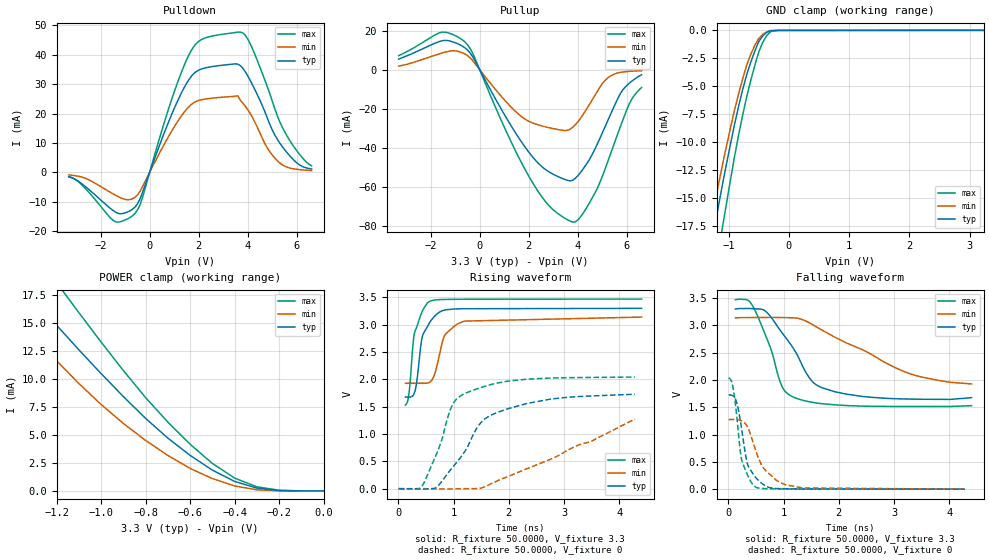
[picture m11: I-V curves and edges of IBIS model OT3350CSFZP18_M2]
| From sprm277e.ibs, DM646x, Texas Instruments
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|   Model Cell OT3350CSFZP18_M2
[Model]   OT3350CSFZP18_M2
Model_type   3-state
Polarity   Non-Inverting
Enable   Active-Low
Cref =  10.0000pF
Rref =  50.0000
Vref =  1.5V
Vmeas =  1.65
C_comp   1.576969p   1.541206p   1.618956p
[Temperature Range]   25   105   0
[Voltage Range]   3.3   3.14   3.47
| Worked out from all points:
|   slope of the pulldown table from 0 to 0.495 V, typ, clamps not added: 44 ohm
|   slope of the pullup table from 0 to 0.495 V, typ, clamps not added: 42.8 ohm
|   GND clamp passes 1 mA (typ) near -0.50 V on its own axis
|   POWER clamp passes 1 mA (typ) near -0.42 V on its own axis
|   rising waveform, R_fixture 50.0000, V_fixture 3.3: 20-80 % time 191ps typ, 250ps min, 163ps max; typ from 1.68 V to 3.3 V
|   rising waveform, R_fixture 50.0000, V_fixture 0: 20-80 % time 815ps typ, 1.73ns min, 454ps max; typ from 0 V to 1.73 V
|   falling waveform, R_fixture 50.0000, V_fixture 3.3: 20-80 % time 603ps typ, 1.42ns min, 389ps max; typ from 3.3 V to 1.68 V
|   falling waveform, R_fixture 50.0000, V_fixture 0: 20-80 % time 210ps typ, 374ps min, 169ps max; typ from 1.73 V to 0 V
[POWER_clamp]
|   voltage   I(typ)   I(min)   I(max)
-3.3V     74.53mA    58.44mA    90.4mA
-1.467V   21.35mA    17.44mA    26.25mA
-1.3V     17.11mA    13.76mA    21.37mA
-1.167V   14.08mA    10.96mA    17.73mA
-1.133V   13.35mA    10.28mA    16.83mA
-1V       10.49mA    7.727mA    13.31mA
-800mV    6.483mA    4.516mA    8.338mA
-600mV    3.176mA    2.013mA    4.168mA
-500mV    1.855mA    1.1mA      2.455mA
-400mV    849.1uA    441.8uA    1.144mA
-300mV    251.7uA    97.47uA    366.8uA
0V        16.5nA     56.13nA    73.26nA
[Pulldown]
|   voltage   I(typ)   I(min)   I(max)
-3.3V     -1.51mA    -878.4uA   -1.475mA
-1.4V     -13.5mA    -7.756mA   -16.81mA
-700mV    -12.57mA   -9.011mA   -14.79mA
-400mV    -9.189mA   -6.568mA   -11.22mA
900mV     19.74mA    14.05mA    24.87mA
1.7V      32.7mA     23.11mA    41.52mA
2.2V      35.39mA    24.85mA    45.53mA
3.6V      36.79mA    25.99mA    47.71mA
4.1V      31.26mA    20mA       43.72mA
5.2V      11.29mA    3.968mA    19.31mA
5.8V      4.81mA     1.296mA    9.68mA
6.6V      1.127mA    609.7uA    2.209mA
[Pullup]
|   voltage   I(typ)   I(min)   I(max)
-3.3V     5.39mA     1.812mA    7.116mA
-1.6V     14.52mA    8.237mA    18.97mA
-600mV    11.14mA    7.957mA    14.14mA
-300mV    6.902mA    4.842mA    8.81mA
1.3V      -29.12mA   -19.41mA   -37.44mA
2.2V      -45.34mA   -27.51mA   -58.77mA
2.9V      -52.9mA    -29.96mA   -70.6mA
3.8V      -56.59mA   -29.42mA   -78.12mA
4.5V      -45.45mA   -17.3mA    -67.66mA
5.2V      -26.73mA   -4.484mA   -47.83mA
6.1V      -6.93mA    -895.9uA   -17.46mA
6.6V      -2.645mA   -585.5uA   -9.164mA
[GND_clamp]
|   voltage   I(typ)   I(min)   I(max)
-3.3V     -90.23mA   -71.94mA   -107.2mA
-1.3V     -19.77mA   -17.29mA   -24.19mA
-1.233V   -17.67mA   -15.49mA   -21.92mA
-1.167V   -15.64mA   -13.72mA   -19.7mA
-1.1V     -13.7mA    -11.97mA   -17.52mA
-900mV    -8.37mA    -7.079mA   -11.23mA
-700mV    -3.966mA   -3.106mA   -5.945mA
-500mV    -1.006mA   -723.8uA   -1.941mA
-366.7mV  -173uA     -140.2uA   -460.9uA
-300mV    -29.43uA   -31.76uA   -99.43uA
-166.7mV  -4.076uA   -4.557uA   -8.063uA
3.233V    -14.06nA   1.378uA    -34.96nA
[Ramp]
| variable   typ   min   max
dV/dt_f  1.0006312/0.62474123n 0.77996615/1.5665136n  1.1807758/0.39522718n
dV/dt_r  1.0444207/0.82282857n 0.78275401/2.2258011n  1.2330064/0.45843701n
R_load = 50
[Rising Waveform]
R_fixture = 50.0000
V_fixture = 3.3
V_fixture_min = 3.14
V_fixture_max = 3.47
|   time   V(typ)   V(min)   V(max)
128.8ps   1.676V     1.928V     1.53V
194.7ps   1.677V     1.929V     1.747V
294ps     1.757V     1.929V     2.847V
336ps     1.964V     1.929V     2.961V
429.8ps   2.756V     1.928V     3.232V
574.4ps   3.05V      1.953V     3.429V
665.6ps   3.164V     2.119V     3.453V
837.5ps   3.268V     2.799V     3.463V
1.197ns   3.293V     3.067V     3.467V
4.402ns   3.3V       3.14V      3.47V
[Rising Waveform]
R_fixture = 50.0000
V_fixture = 0
V_fixture_min = 0
V_fixture_max = 0
|   time   V(typ)   V(min)   V(max)
8.072ps   17.64uV    17.18uV    19.99uV
428.3ps   -8.284mV   14.33uV    42.96mV
687ps     22.56mV    -1.575mV   622mV
965.9ps   369.3mV    -4.262mV   1.503V
1.053ns   475.1mV    -2.583mV   1.637V
1.201ns   675.7mV    -1.005mV   1.739V
1.519ns   1.234V     17.47mV    1.859V
1.971ns   1.458V     217mV      1.965V
2.879ns   1.654V     596mV      2.028V
4.282ns   1.728V     1.275V     2.043V
[Falling Waveform]
R_fixture = 50.0000
V_fixture = 3.3
V_fixture_min = 3.14
V_fixture_max = 3.47
|   time   V(typ)   V(min)   V(max)
128.8ps   3.3V       3.14V      3.47V
337.5ps   3.31V      3.143V     3.469V
433.7ps   3.307V     3.144V     3.371V
671.7ps   3.261V     3.145V     2.826V
968.6ps   2.871V     3.143V     1.892V
1.177ns   2.58V      3.139V     1.687V
1.517ns   1.977V     3.019V     1.591V
1.923ns   1.787V     2.787V     1.545V
3.294ns   1.65V      2.112V     1.515V
4.402ns   1.676V     1.928V     1.53V
[Falling Waveform]
R_fixture = 50.0000
V_fixture = 0
V_fixture_min = 0
V_fixture_max = 0
|   time   V(typ)   V(min)   V(max)
8.072ps   1.728V     1.275V     2.043V
95.7ps    1.7V       1.277V     1.808V
165.3ps   1.539V     1.272V     1.234V
217.1ps   1.267V     1.261V     699.4mV
247.5ps   1.069V     1.249V     519.5mV
348.4ps   463.7mV    1.139V     262.5mV
500.5ps   209.3mV    697.7mV    34.93mV
653.7ps   72.17mV    367.2mV    10.43mV
1.033ns   6.697mV    80.88mV    3.604mV
4.282ns   17.64uV    17.18uV    19.99uV
